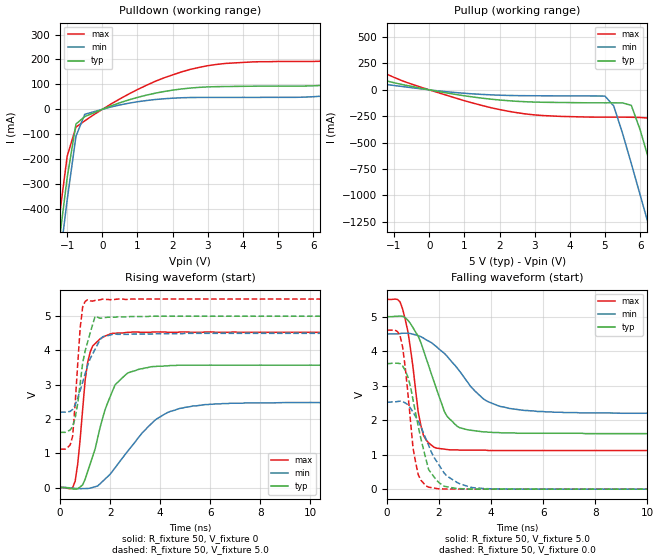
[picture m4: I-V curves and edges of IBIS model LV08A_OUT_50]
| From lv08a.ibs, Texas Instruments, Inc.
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|   Model LV08A_OUT_50
[Model]   LV08A_OUT_50
Model_type  Output
Polarity   Non-Inverting
Vmeas = 2.50v
Cref = 15pf
| variable   typ   min   max
C_comp   4.62pf   3.47pf   5.77pf
[Temperature Range]   25   85   -40
[Voltage Range]   5.0   4.5   5.5
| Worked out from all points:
|   slope of the pulldown table from 0 to 0.75 V, typ, clamps not added: 19.9 ohm
|   slope of the pullup table from 0 to 0.75 V, typ, clamps not added: 17.2 ohm
|   rising waveform, R_fixture 50, V_fixture 0: 20-80 % time 903ps typ, 1.72ns min, 363ps max; typ from 0 V to 3.57 V
|   falling waveform, R_fixture 50, V_fixture 5.0: 20-80 % time 927ps typ, 1.61ns min, 475ps max; typ from 5 V to 1.61 V
|   rising waveform, R_fixture 50, V_fixture 5.0: 20-80 % time 465ps typ, 677ps min, 245ps max; typ from 1.61 V to 5 V
|   falling waveform, R_fixture 50, V_fixture 0.0: 20-80 % time 627ps typ, 1ns min, 392ps max; typ from 3.64 V to 0 V
[Pulldown]
|   Voltage   I(typ)   I(min)   I(max)
-5V       -5.14A     -5.22A     -5.05A
-1.5V     -853mA     -945mA     -756mA
-1.25V    -557mA     -649mA     -461mA
-1V       -274mA     -363mA     -188mA
-750mV    -58.9mA    -108mA     -71.3mA
-500mV    -29.2mA    -20mA      -46.2mA
0V        -3.33nA    -3.4nA     -3.57nA
1.25V     56.7mA     35.2mA     96mA
2.5V      85.3mA     47.3mA     160mA
3.5V      91.4mA     47.8mA     184mA
6.75V     103mA      58.5mA     199mA
10V       179mA      107mA      329mA
[Pullup]
|   Voltage   I(typ)   I(min)   I(max)
-5V       310mA      167mA      586mA
-3.5V     252mA      143mA      464mA
-750mV    48.6mA     30.8mA     83.5mA
1.5V      -78.8mA    -43.4mA    -148mA
5V        -123mA     -58.9mA    -259mA
5.25V     -123mA     -153mA     -259mA
5.75V     -147mA     -699mA     -260mA
6.25V     -664mA     -1.29A     -268mA
6.5V      -960mA     -1.6A      -403mA
6.75V     -1.26A     -1.9A      -685mA
7.25V     -1.87A     -2.51A     -1.28A
10V       -5.25A     -5.89A     -4.66A
[Ramp]
| variable   typ   min   max
dV/dt_r   2.15E+00/8.50E-10   1.50E+00/1.76E-09   2.72E+00/3.42E-10
dV/dt_f   2.05E+00/9.19E-10   1.39E+00/1.59E-09   2.64E+00/5.26E-10
R_load = 50
[Rising Waveform]
R_fixture = 50
V_fixture = 0
|   Time   V(typ)   V(min)   V(max)
0s        0V         0V         0V
600ps     -48.3mV    -27.4mV    185mV
800ps     18.3mV     -32.7mV    1.41V
1ns       245mV      -30.5mV    3.14V
1.2ns     687mV      -19mV      3.95V
2.1ns     2.83V      484mV      4.5V
2.7ns     3.34V      1.06V      4.53V
3.8ns     3.53V      1.97V      4.54V
5.3ns     3.57V      2.38V      4.53V
25ns      3.57V      2.48V      4.53V
[Falling Waveform]
R_fixture = 50
V_fixture = 5.0
V_fixture_min = 4.5
V_fixture_max = 5.5
|   Time   V(typ)   V(min)   V(max)
0s        5V         4.5V       5.5V
600ps     5.01V      4.52V      5.22V
800ps     4.9V       4.52V      4.58V
1.3ns     4.25V      4.42V      1.85V
1.9ns     2.91V      4.13V      1.19V
2.3ns     2.12V      3.86V      1.15V
2.8ns     1.78V      3.41V      1.13V
3.8ns     1.66V      2.57V      1.13V
5.3ns     1.62V      2.28V      1.12V
25ns      1.61V      2.2V       1.12V
[Rising Waveform]
R_fixture = 50
V_fixture = 5.0
V_fixture_min = 4.5
V_fixture_max = 5.5
|   Time   V(typ)   V(min)   V(max)
0s        1.61V      2.2V       1.12V
400ps     1.68V      2.22V      1.24V
500ps     1.78V      2.28V      1.5V
800ps     3.03V      2.83V      4.65V
900ps     3.63V      3.07V      5.27V
1.1ns     4.25V      3.57V      5.48V
1.4ns     5V         4.04V      5.46V
1.7ns     4.95V      4.4V       5.5V
2.2ns     4.97V      4.48V      5.49V
25ns      5V         4.5V       5.5V
[Falling Waveform]
R_fixture = 50
V_fixture = 0.0
|   Time   V(typ)   V(min)   V(max)
0s        3.64V      2.52V      4.61V
500ps     3.64V      2.55V      4.45V
800ps     3.26V      2.45V      2.8V
1ns       2.59V      2.23V      1.19V
1.1ns     2.2V       2.1V       777mV
1.3ns     1.47V      1.82V      262mV
1.6ns     568mV      1.27V      57.6mV
2.3ns     69.7mV     382mV      5.57mV
3.7ns     4.92mV     19.4mV     1.1mV
25ns      8.88uV     2.8uV      9.54uV
